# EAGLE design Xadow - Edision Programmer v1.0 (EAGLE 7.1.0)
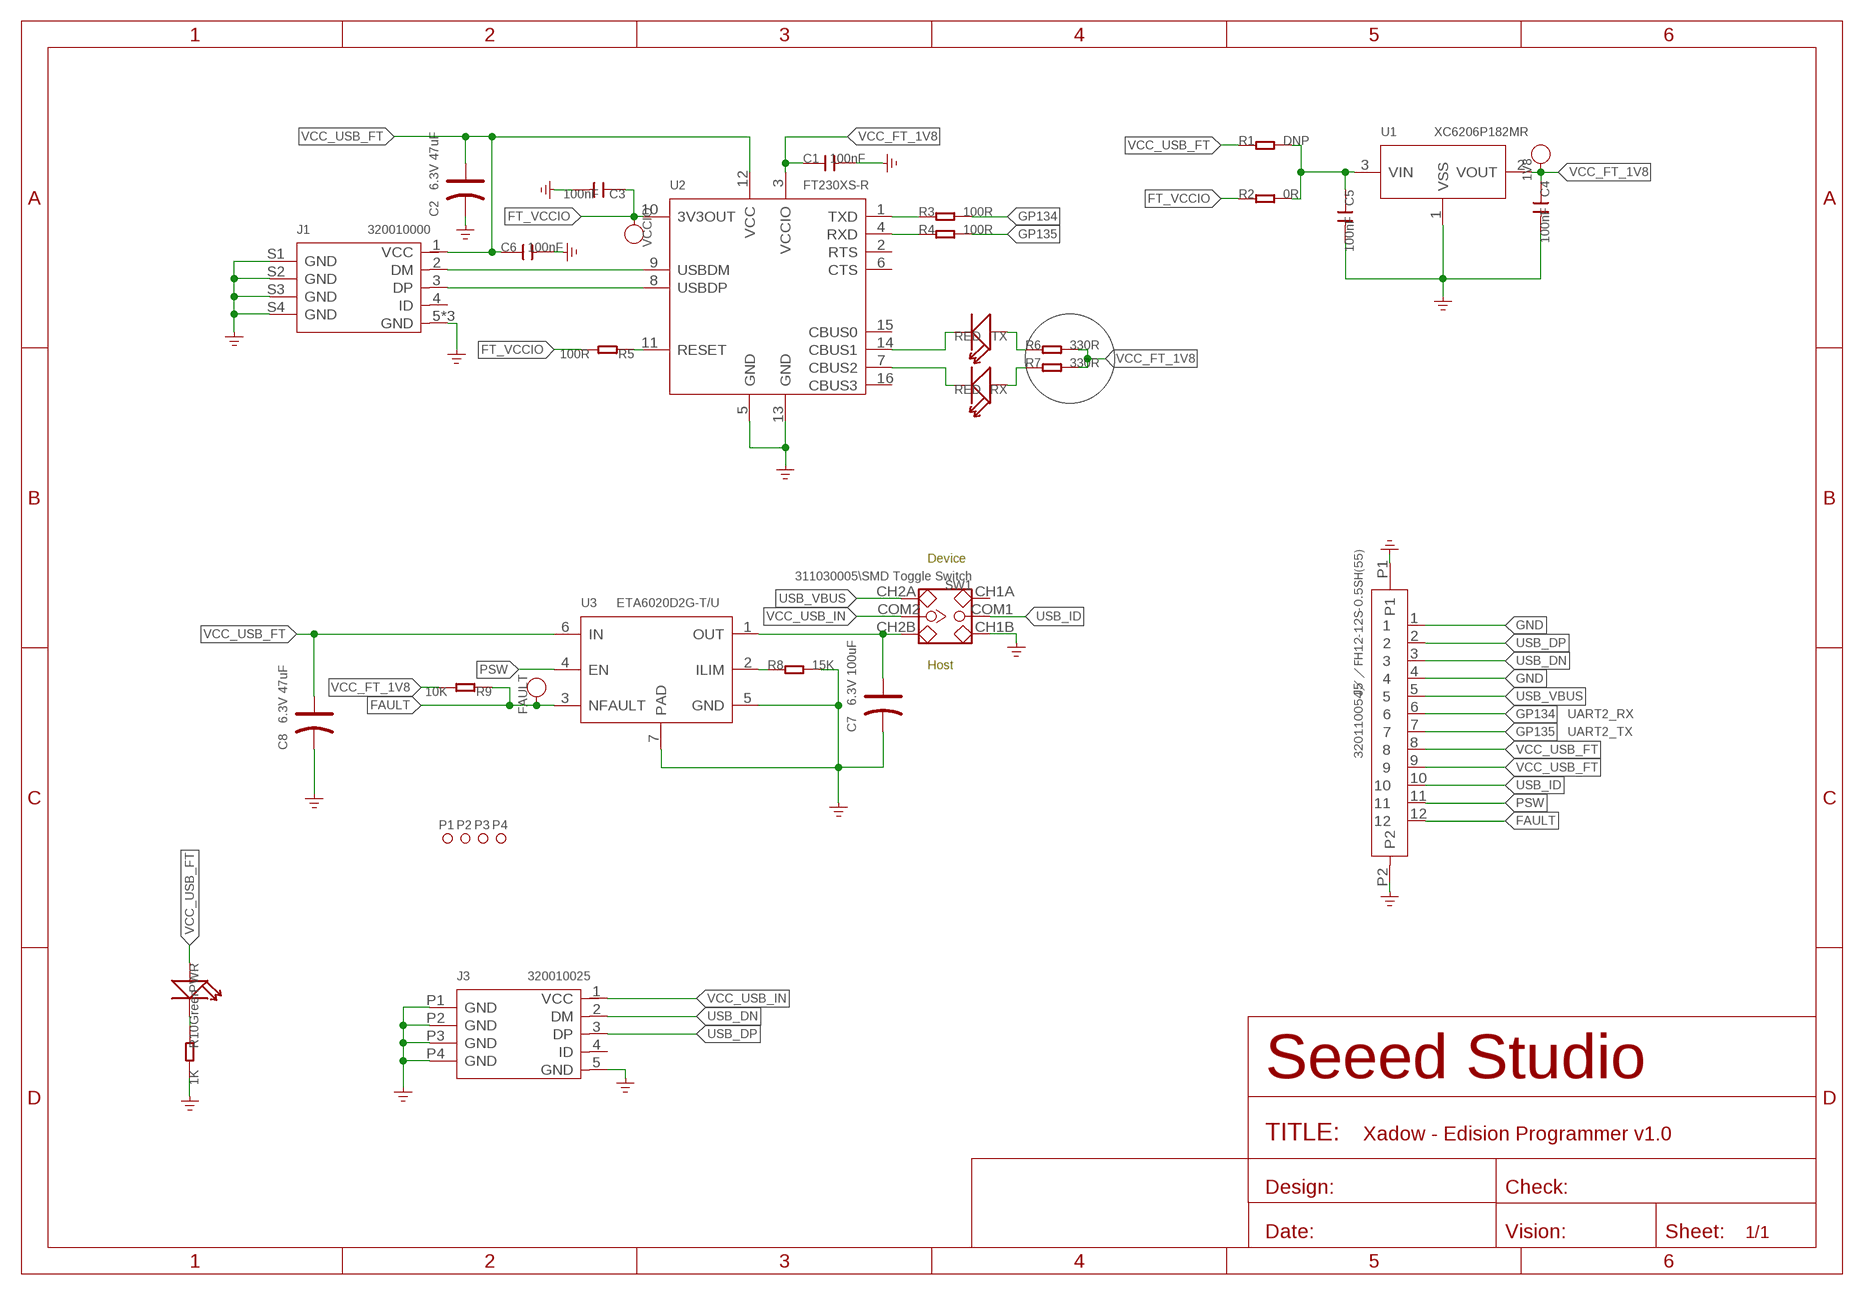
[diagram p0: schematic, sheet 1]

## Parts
1V8  DNP  PAD-TEST-POINT'4545'  [TP-D45MIL]
C1  100nF  C-0402  [C0402]
C2  6.3V 47uF  CAP-POLAR-AVX-A  [AVX-A]
C3  100nF  C-0402  [C0402]
C4  100nF  C-0402  [C0402]
C5  100nF  C-0402  [C0402]
C6  100nF  C-0402  [C0402]
C7  6.3V 100uF  CAP-POLAR-AVX-B  [AVX-B]
C8  6.3V 47uF  CAP-POLAR-AVX-A  [AVX-A]
FAULT  DNP  PAD-TEST-POINT'4545'  [TP-D45MIL]
J1  320010000  USB-MICRO-5P'5+4P'  [5+4P-SMD-0.65-B]
J3  320010025  USB-MICRO-5P'ALX-MC-5F-036'  [5+2P-SMD-0.65-AB]
J5  320110054／／FH12-12S-0.5SH(55)  FPC052002-12LT-FH12-12S-0.5SH  [12P-0.5-NEW]
P1  PAD-MARK'ANNULAR'  [ROUND-MARK-1.0]
P2  PAD-MARK'ANNULAR'  [ROUND-MARK-1.0]
P3  PAD-MARK'ANNULAR'  [ROUND-MARK-1.0]
P4  PAD-MARK'ANNULAR'  [ROUND-MARK-1.0]
PWR  Green  LED'0603'  [LED-0603]
R1  DNP  R-0402  [R0402]
R2  0R  R-0402  [R0402]
R3  100R  R-0402  [R0402]
R4  100R  R-0402  [R0402]
R5  100R  R-0402  [R0402]
R6  330R  R-0402  [R0402]
R7  330R  R-0402  [R0402]
R8  15K  R-0402  [R0402]
R9  10K  R-0402  [R0402]
R10  1K  R-0402  [R0402]
RX  RED  LED'0603'  [LED-0603]
SW1  311030005\\SMD Toggle Switch  SWITCH-2CH-6P-SMD  [6P-SMD-2CH-2.54-3.5X7.2]
TX  RED  LED'0603'  [LED-0603]
U1  XC6206P182MR  PMIC-XC6206PMR  [SOT-23]
U2  FT230XS-R  FT230XS  [SSOP16]
U3  ETA6020D2G-T/U  ETA6020  [6P-0.65-L2*W2*H0.75MM]
VCCIO  DNP  PAD-TEST-POINT'4545'  [TP-D45MIL]

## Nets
FAULT: FAULT.T J5.12 R9.1 U3.3(NFAULT)
FT_RX: R4.1 U2.4(RXD)
FT_TX: R3.1 U2.1(TXD)
FT_VCCIO: C3.1 R2.1 R5.2 U2.10(3V3OUT) VCCIO.T
GND: C1.2 C2.- C3.2 C4.2 C5.2 C6.2 C7.- C8.- J1.5(GND) J1.S1(GND) J1.S2(GND) J1.S3(GND) J1.S4(GND) J1.S5(GND) J1.S6(GND) J3.5(GND) J3.P1(GND) J3.P2(GND) J3.P3(GND) J3.P4(GND) J5.1 J5.4 J5.P1 J5.P2 R8.2 R10.2 SW1.CH1B U1.1(VSS) U2.5(GND) U2.13(GND) U3.5(GND) U3.7(PAD) ; supply symbol labelled GND_POWER
GP134: J5.6 R3.2
GP135: J5.7 R4.2
N$1: J1.2(DM) U2.9(USBDM)
N$2: J1.3(DP) U2.8(USBDP)
N$3: PWR.- R10.1
N$5: R5.1 U2.11(RESET)
N$22: TX.- U2.14(CBUS1)
N$41: RX.- U2.7(CBUS2)
N$52: R6.1 TX.+
N$54: R7.1 RX.+
N$56: C5.1 R1.2 R2.2 U1.3(VIN)
N$75: C7.+ SW1.CH2B U3.1(OUT)
N$77: R8.1 U3.2(ILIM)
PSW: J5.11 U3.4(EN)
USB_DN: J3.2(DM) J5.3
USB_DP: J3.3(DP) J5.2
USB_ID: J5.10 SW1.COM1
USB_VBUS: J5.5 SW1.CH2A
VCC_FT_1V8: 1V8.T C1.1 C4.1 R6.2 R7.2 R9.2 U1.2(VOUT) U2.3(VCCIO)
VCC_USB_FT: C2.+ C6.1 C8.+ J1.1(VCC) J5.8 J5.9 PWR.+ R1.1 U2.12(VCC) U3.6(IN)
VCC_USB_IN: J3.1(VCC) SW1.COM2
Unconnected: J1.4(ID) J3.4(ID) SW1.CH1A U2.2(RTS) U2.6(CTS) U2.15(CBUS0) U2.16(CBUS3)

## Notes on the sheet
- Device
- Host
- UART2_RX
- UART2_TX

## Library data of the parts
1V8 FAULT VCCIO = Discrete-new:PAD-TEST-POINT; PARTNO: DNP
C1 C3-C6 = Discrete:C*: Ceramic Capacitors
C2 C7 C8 = Discrete-new:CAP-POLAR: Electrolytic Capacitors,Tantalum Capacitors and Super Capacitors
J1 = Connector:USB-MICRO-5P: 5+4P-SMD-0.65-B:320010000 5+2P-SMD-0.65-AB:340032001
J3 = Connector-new:USB-MICRO-5P: 5+4P-SMD-0.65-B:320010000;5+2P-SMD-0.65-AB:340032001
J5 = template:FPC052002-12LT
P1-P4 = Discrete-new:PAD-MARK; PARTNO: DNP
PWR RX TX = Discrete:LED*
R1-R10 = Discrete:R*
SW1 = Discrete:SWITCH-2CH-6P
U1 = IC-NEW:PMIC-XC6206P: LOW ESR Cap.Compatible Positive Voltage Regulators
U2 = template:FT230XS: The FT230X is a USB to serial UART
U3 = template:ETA6020: Precision Load Switch with Adjustable Current Limit

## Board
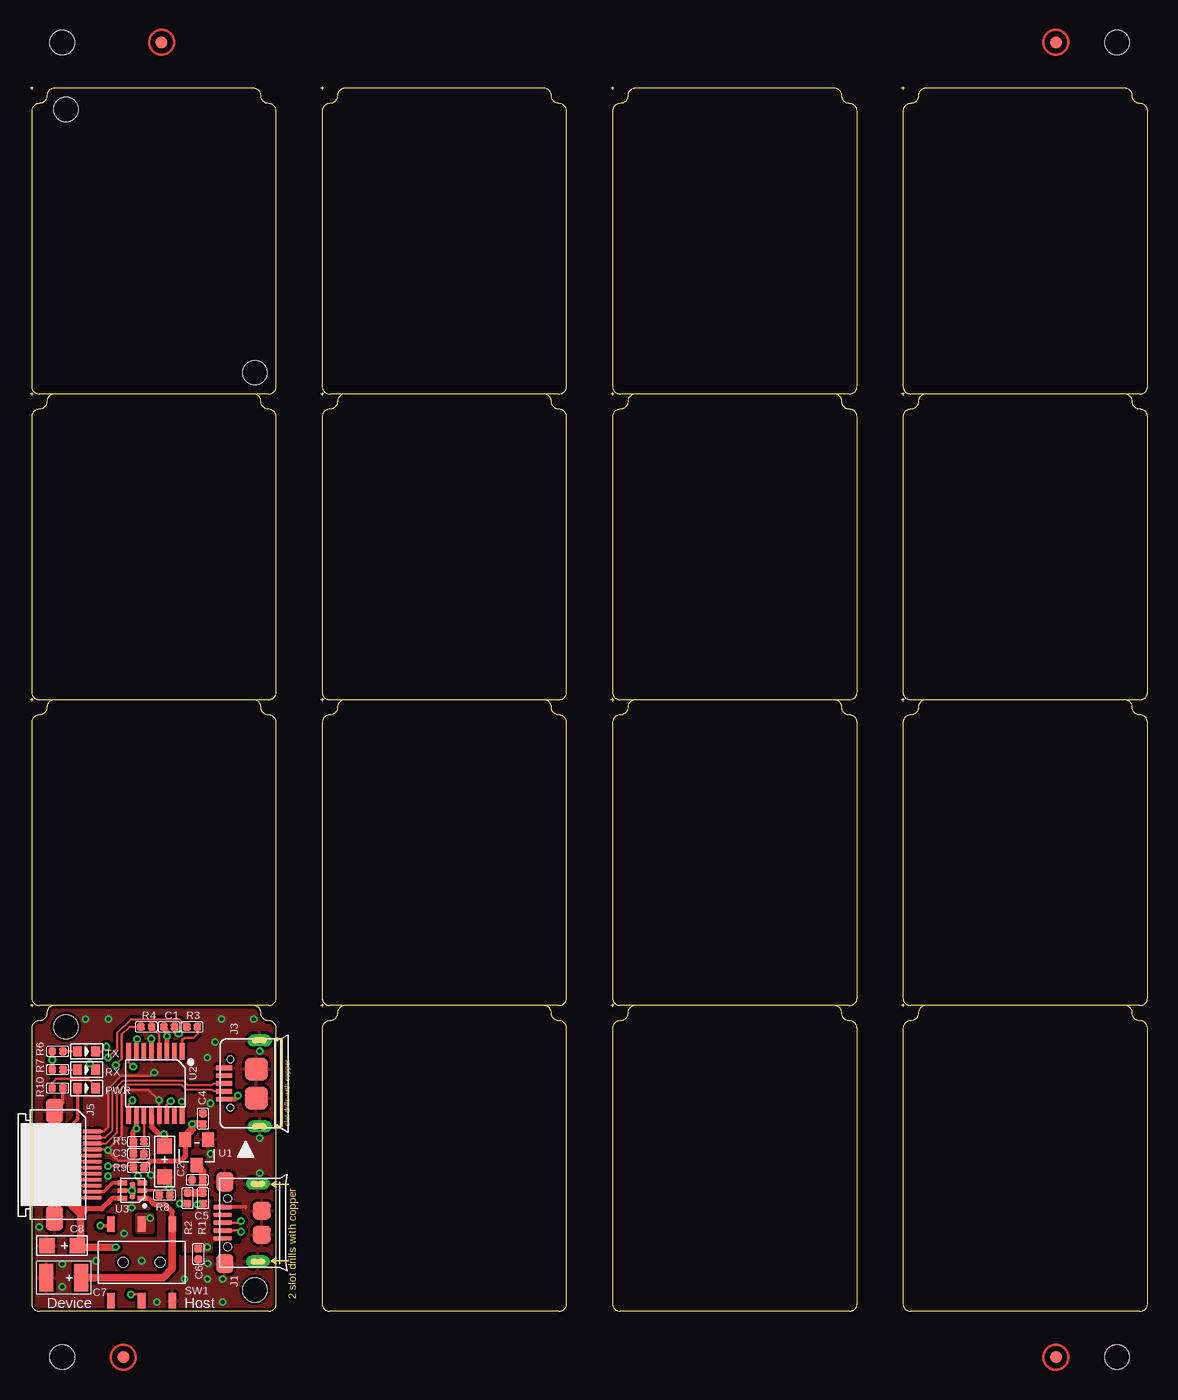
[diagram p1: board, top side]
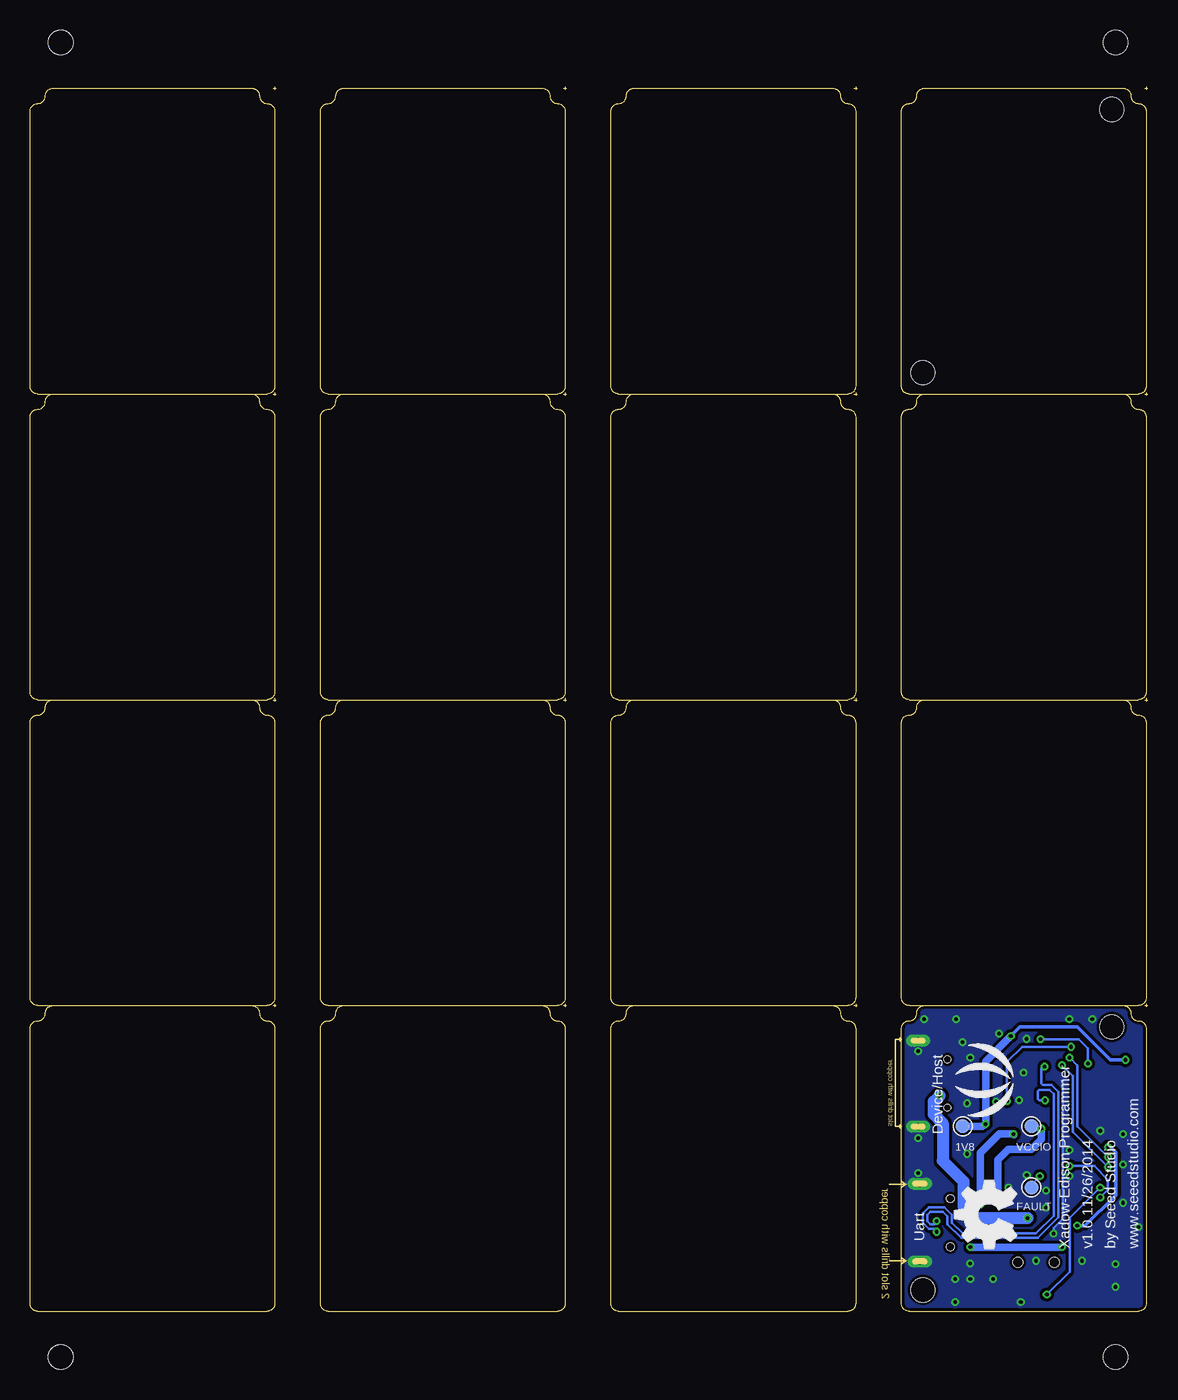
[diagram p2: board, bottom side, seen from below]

Size 92.84 x 101.73 mm. Coordinates in mm from the lower left corner, seen from the top.
Outline: 248 segments
Copper layers (1*16): Top 0.035mm / dielectric 1.5mm / Bottom 0.035mm
Design rules "SeeedStudio_2layer_DRU_no_angle_20140221 *": minimum track width 5mil, minimum drill 12mil, track to track 6mil, track to pad 6mil, pad to pad 6mil, via to via 6mil, smd to smd 0mil, copper to edge 10mil, drill to drill 10mil, minimum pad ring 10mil, minimum via ring 6mil, stop-mask expansion 2mil, vias tented up to drill 100mil, thermal gap 10mil
Holes 2 mm at 2.98,23.62 18.67,1.78 2.98,99.82 18.67,77.98
Holes 2.03 mm at 2.67,105.41 90.3,105.41 2.67,-3.81 90.3,-3.81

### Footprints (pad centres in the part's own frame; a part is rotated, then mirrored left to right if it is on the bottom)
TP-D45MIL = smd 1.143 x 1.143: T 0,0
C0402 = smd 0.635 x 0.635: 1 -0.445,0; 2 0.445,0
AVX-A = smd 1.27 x 1.27: + -1.27,0; - 1.27,0
AVX-B = smd 1.143 x 2.286: + -1.46,0; - 1.46,0
5+4P-SMD-0.65-B = smd 0.381 x 1.524: 1 -1.3,-0.25; 2 -0.65,-0.25; 3 0,-0.25; 4 0.65,-0.25; 5 1.3,-0.25 | smd 1.6 x 1.397: S1 -3.4,-0.427; S6 3.4,-0.427 | drill 0.508 pad 1.016 long: S2 -3.226,-3.175; S5 3.226,-3.175 | smd 1.5 x 1.5: S3 -1,-3.5; S4 1,-3.5 | hole 0.635: -2,-0.65; 2,-0.65
5+2P-SMD-0.65-AB = smd 0.4 x 1.35: 1 -1.3,2.675; 2 -0.65,2.675; 3 0,2.675; 4 0.65,2.675; 5 1.3,2.675 | smd 1.9 x 1.9: P1 -1.2,0; P2 1.2,0 | drill 0.508 pad 1.016 long: P3 -3.575,-0.265; P4 3.575,-0.265 | hole 0.55: -2,2.15; 2,2.15
12P-0.5-NEW = smd 0.3 x 1.6: 1 -2.75,3.127; 2 -2.25,3.127; 3 -1.75,3.127; 4 -1.25,3.127; 5 -0.75,3.127; 6 -0.25,3.127; 7 0.25,3.127; 8 0.75,3.127; 9 1.25,3.127; 10 1.75,3.127; 11 2.25,3.127; 12 2.75,3.127 | smd 2.032 x 1.397: P1 -4.445,0; P2 4.445,0
ROUND-MARK-1.0 = smd 1.016 x 1.016: P$1 0,0
LED-0603 = smd 0.762 x 0.889: + -0.762,0; - 0.762,0
R0402 = smd 0.635 x 0.635: 1 -0.445,0; 2 0.445,0
6P-SMD-2CH-2.54-3.5X7.2 = smd 1.27 x 0.635: CH1A -3.175,2.54; CH1B -3.175,-2.54; CH2A 3.175,2.54; CH2B 3.175,-2.54; COM1 -3.175,0; COM2 3.175,0 | hole 0.813: 0,1.524; 0,-1.524
SOT-23 = smd 1.016 x 1.2: 1 -0.95,-1.06; 2 0.95,-1.06; 3 0,1.06
SSOP16 = smd 0.381 x 1.397: 1 -2.223,-2.667; 2 -1.587,-2.667; 3 -0.953,-2.667; 4 -0.318,-2.667; 5 0.318,-2.667; 6 0.953,-2.667; 7 1.587,-2.667; 8 2.223,-2.667; 9 2.223,2.667; 10 1.587,2.667; 11 0.953,2.667; 12 0.318,2.667; 13 -0.318,2.667; 14 -0.953,2.667; 15 -1.587,2.667; 16 -2.223,2.667
6P-0.65-L2*W2*H0.75MM = smd 0.4 x 0.8: 1 -0.65,-0.827; 2 0,-0.827; 3 0.65,-0.827; 4 0.65,0.827; 5 0,0.827; 6 -0.65,0.827 | smd 1.4 x 0.5: 7 0,0

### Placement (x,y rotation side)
1V8  15.37,15.37 0 bottom
C1  11.56,23.62 0 top
C2  11.18,12.45 270 top
C3  9.02,13.08 0 top
C4  14.35,16 90 top
C5  13.91,10.92 180 top
C6  13.97,4.76 270 top
C7  2.79,2.79 180 top
C8  2.67,5.46 180 top
FAULT  9.65,10.29 0 bottom
J1  15.75,7.37 90 top
J3  18.8,18.92 90 top
J5  2.03,12.19 270 top
P1  not placed on the board
P2  not placed on the board
P3  not placed on the board
P4  not placed on the board
PWR  4.7,18.54 0 top
R1  14.35,9.4 90 top
R2  13.08,9.4 90 top
R3  13.46,23.62 180 top
R4  9.65,23.62 180 top
R5  9.02,14.1 180 top
R6  2.29,21.59 180 top
R7  2.29,20.07 180 top
R8  11.18,9.65 0 top
R9  9.02,11.94 0 top
R10  2.29,18.54 0 top
RX  4.7,20.07 0 top
SW1  9.27,4.06 90 top
TX  4.7,21.59 0 top
U1  13.84,13.21 180 top
U2  10.41,18.92 180 top
U3  8.51,10.03 90 top
U$39  [LOGO_SILK]  12.83,19.18 90 bottom
U$80  [OSHW_FILLX200_NOTEXT]  10.92,5.21 90 bottom
VCCIO  9.65,15.37 0 bottom

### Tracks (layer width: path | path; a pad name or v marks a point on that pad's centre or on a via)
FAULT  (via drill 0.3 pad 0.64)
  Top 0.203: v6.48,12.07 8.45,12.07 R9.1 8.95,11.56 v8.95,11.24 8.95,10.99 9.14,10.8 9.22,10.8 U3.3 | J5.12 3.96,9.44 v3.94,9.46
  Top 0.305: 8.64,11.88 8.64,12 R9.1
  Bottom 0.203: v6.48,12.07 4.45,12.07 3.3,10.92 3.3,10.1 v3.94,9.46 | 9.65,10.61 9.59,10.61 v8.95,11.24
  Bottom 0.305: FAULT.T 9.65,10.61
FT_RX
  Top 0.203: U2.4 10.73,22.99 R4.1
FT_TX
  Top 0.203: U2.1 12.64,22.54 12.83,22.73 13.59,22.73 13.91,23.05 R3.1
FT_VCCIO  (via drill 0.3 pad 0.64)
  Top 0.406: R5.2 8.57,14.92 v8.83,15.18 U2.10
  Top 0.61: R2.1 12.83,8.95 | C3.1 R5.2
  Top 0.635: 12.83,8.95 v12.45,8.95
  Bottom 0.406: v8.83,15.18 9.46,15.18 VCCIO.T
  Bottom 0.61: v8.83,15.18 8.83,14.29 9.65,13.46 11.56,13.46
  Bottom 0.635: v12.45,8.95 12.45,12.57 11.56,13.46
GND  (via drill 0.3 pad 0.64)
  Top 0.203: J5.1 6.12,14.94 6.48,15.3 6.48,18.48 7.56,19.56 10.03,19.56 v10.31,19.84 | J5.4 6.46,13.44 7.62,14.61 7.62,17.97 8.06,18.41 9.83,18.41 v10.69,17.55 10.73,17.51 U2.13 | C3.2 9.34,12.95 9.34,12.89 8.95,12.51 7.3,12.51 7.11,12.7
  Top 0.305: J1.5 17.88,8.67 17.91,8.64 | R10.2 2.73,17.34 J5.P1 | 6.46,13.44 6.46,13.36 7.11,12.7
  Top 0.406: C1.2 12,23.42 v12.34,23.08 | U2.5 10.1,22.59 v10.06,22.63
  Bottom 0.203: v7.81,6.46 7.81,6.92 7.05,7.68 7.05,19.05 7.14,19.14
  other vias: 8.45,8.62 19.08,11.48 16,2.67 14.76,3.96 14.73,2.67 2.67,3.94 10.54,0.76 2.67,2.03 16,0.76 2.03,9.02 2.03,12.19 2.03,14.73 15.37,22.35 14.73,21.08 14.99,17.27 12.6,17.42 19.08,14.38 19.08,21.62 4.6,24.28 6.5,24.28 15.9,24.28 18.57,24.28 8.45,10.02 6.48,11.23 10.03,11.3 11.56,10.29 0.76,6.99 6.48,13.4 3.94,14.99 14.99,13.08 12.83,2.67 5.46,4.19 9.27,4.19
  pour Bottom (isolate 0.254, rank 6, no thermals): -0.51,26.16 21.08,26.16 21.08,-0.51 -0.51,-0.51
  pour Top (isolate 0.254, rank 6): -0.51,26.16 21.08,26.16 21.08,-0.51 -0.51,-0.51
GP134  (via drill 0.3 pad 0.64)
  Top 0.203: R3.2 12.38,24.26 8.38,24.26 7.24,23.11 7.24,21.84 v6.48,21.08 | J5.6 3.69,12.44 v3.3,12.83
  Bottom 0.203: v6.48,21.08 5.84,20.45 5.84,15.37 v3.3,12.83
GP135  (via drill 0.3 pad 0.64)
  Top 0.203: R4.2 8.26,23.62 7.62,22.99 7.62,20.96 v7.11,20.45 | J5.7 3.36,11.94 v3.3,12
  Bottom 0.203: v7.11,20.45 6.22,19.56 6.22,14.92 v3.3,12
N$1  (via drill 0.3 pad 0.64)
  Top 0.203: U2.9 8.19,17.21 v8.51,17.53 | J1.2 17.41,6.72 v17.53,6.6
  Bottom 0.203: v8.51,17.53 9.02,17.53 9.14,17.65 9.14,18.29 9.02,18.41 8.17,18.41 7.81,18.06 7.81,7.94 9.27,6.48 15.37,6.48 16.26,7.37 16.26,8 16.89,8.64 18.16,8.64 18.67,8.13 18.67,7.37 18.16,6.86 17.78,6.86 v17.53,6.6
N$2  (via drill 0.3 pad 0.64)
  Top 0.203: U2.8 8.19,20.69 v8.56,20.32 | J1.3 17.4,7.37 v17.53,7.49
  Bottom 0.203: v17.53,7.49 17.78,7.24 18.03,7.24 18.29,7.49 18.29,8 18.03,8.25 17.02,8.25 16.64,7.87 16.64,7.24 15.49,6.1 9.14,6.1 7.43,7.81 7.43,18.22 8,18.8 8.7,18.8 8.83,18.92 8.83,20.19 8.7,20.32 v8.56,20.32
N$3
  Top 0.203: PWR.- 5.46,18.67 4.83,19.3 2.16,19.3 1.84,18.99 R10.1
N$5
  Top 0.203: U2.11 R5.1
N$22  (via drill 0.3 pad 0.64)
  Top 0.203: U2.14 11.37,17.14 v11.68,17.46 | TX.- 5.97,21.59 v6.35,21.97
  Bottom 0.203: v11.68,17.46 11.68,20.7 10.41,21.97 v6.35,21.97
N$41  (via drill 0.3 pad 0.64)
  Top 0.203: U2.7 8.83,22.54 v8.89,22.61 | RX.- 5.46,20.19 5.33,20.19 v4.95,20.57
  Bottom 0.203: v8.89,22.61 5.72,22.61 4.95,21.84 v4.95,20.57
N$52
  Top 0.203: R6.1 TX.+
N$54
  Top 0.203: RX.+ R7.1
N$56
  Top 0.61: R2.2 R1.2 C5.1 14.35,11.64 U1.3 13.84,11.94
N$75
  Top 0.406: U3.1 9.79,9.38 10.29,8.89 11.18,8.89 11.81,8.25 SW1.CH2B
  Top 0.61: SW1.CH2B 11.81,3.56 11.05,2.79 C7.+
N$77
  Top 0.203: U3.2 10.35,10.03 R8.1
PSW
  Top 0.305: J5.11 6.13,9.94 6.87,10.68 U3.4
USB_DN
  Top 0.152: J3.2 15.26,18.27 15.11,18.41 12.95,18.41 12.57,18.8 7.87,18.8 7.24,18.16 7.24,14.86 6.32,13.94 J5.3
USB_DP
  Top 0.152: J3.3 15.24,18.92 15.11,18.8 13.08,18.8 12.7,19.18 7.75,19.18 6.86,18.29 6.86,15.04 6.26,14.44 J5.2
USB_ID  (via drill 0.3 pad 0.64)
  Top 0.203: J5.10 4.09,10.44 v3.94,10.29 | 9.27,0.76 SW1.COM1 9.27,1.14 9.02,1.4 v8.38,1.4
  Bottom 0.203: v3.94,10.29 6.48,7.75 6.48,3.3 v8.38,1.4
USB_VBUS  (via drill 0.3 pad 0.64)
  Top 0.203: 6.6,7.11 SW1.CH2A
  Top 0.305: J5.5 4.14,12.94 3.43,13.65 v3.3,13.65 | v5.84,7.11 6.86,7.11 SW1.CH2A
  Bottom 0.305: v3.3,13.65 3.11,13.65 2.67,13.21 2.67,9.65 5.21,7.11 v5.84,7.11
VCC_FT_1V8  (via drill 0.3 pad 0.64)
  Top 0.305: R6.2 v1.84,20.89 R7.2
  Top 0.406: C1.1 11.11,23.5 11.37,23.24 v11.37,22.86 U2.3 | U1.2 12.89,12.89 12.45,12.45 9.97,12.45 R9.2
  Top 0.61: U1.2 12.89,14.54 13.46,15.11 13.46,15.49 | 13.46,15.49 v13.46,15.56 | C4.1 13.53,15.56 13.46,15.49
  Bottom 0.305: v1.84,20.89 3.11,20.89 5.84,23.62 10.6,23.62 v11.37,22.86
  Bottom 0.61: v13.46,15.56 13.46,15.62 | 1V8.T 13.72,15.37 13.46,15.62 | 13.46,15.62 13.46,20.77 v11.37,22.86
VCC_USB_FT  (via drill 0.3 pad 0.64)
  Top 0.305: PWR.+ 3.94,16 2.67,14.73 2.67,10.92 2.69,10.94 3.07,10.94 | J5.9 4.04,10.94 | 4.04,10.94 3.94,10.94 | J5.8 4.08,11.44 3.94,11.3 3.94,11.05 | 3.94,11.05 3.94,10.94 | 3.94,10.94 3.07,10.94 | 3.07,10.94 2.79,10.67 | 4.04,10.94 3.94,11.05
  Top 0.406: U2.12 10.1,15.3 10.67,14.73 v11.12,14.73 | U3.6 6.84,9.38 5.97,8.51 4.7,8.51 | 4.7,8.51 3.81,8.51 3.78,8.48 | 4.7,8.51 4.19,8
  Top 0.61: C2.+ 11.18,14.68 v11.12,14.73 | 4.06,5.33 C8.+ | 2.67,10.92 2.67,9.59 3.78,8.48 4.19,8.07 4.19,8 4.19,5.46 4.06,5.33 | v7.11,5.33 4.06,5.33
  Top 0.635: 14.35,8.89 13.91,8.89 v13.89,8.88
  Bottom 0.61: v7.11,5.33 v14.73,5.33
  Bottom 0.635: 11.12,14.66 v11.12,14.73 12.32,14.73 13.89,13.16 v13.89,8.88
  pour Top (isolate 0.254, no thermals): 16.89,5.84 15.37,5.84 15.11,5.71 15.11,5.08 14.99,4.95 12.83,4.95 12.7,5.08 12.7,8.13 12.83,8.25 13.72,8.25 13.84,8.38 13.84,9.14 13.97,9.27 14.86,9.27 14.99,9.14 14.99,6.35 15.11,6.22 16.89,6.22
VCC_USB_IN  (via drill 0.3 pad 0.64)
  Top 0.406: v17.27,17.91 16.99,17.62 J3.1
  Bottom 1.016: v17.27,17.91 17.78,17.4 17.78,16.38 17.02,15.62 17.02,12.51 15.3,10.8 15.3,8.7 14.35,7.75 v9.97,7.75
  pour Top (isolate 0.254, no thermals): 9.02,8.13 10.03,8.13 arc-90 10.29,7.87 10.29,6.73 arc-90 10.03,6.48 9.02,6.48 arc-90 8.76,6.73 8.76,7.87 arc-90

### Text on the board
tPlace: Device | Host
bPlace: Device/Host | Uart | www.seeedstudio.com | by Seeed Studio | v1.0 11/26/2014 | Xadow-Edison Programmer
